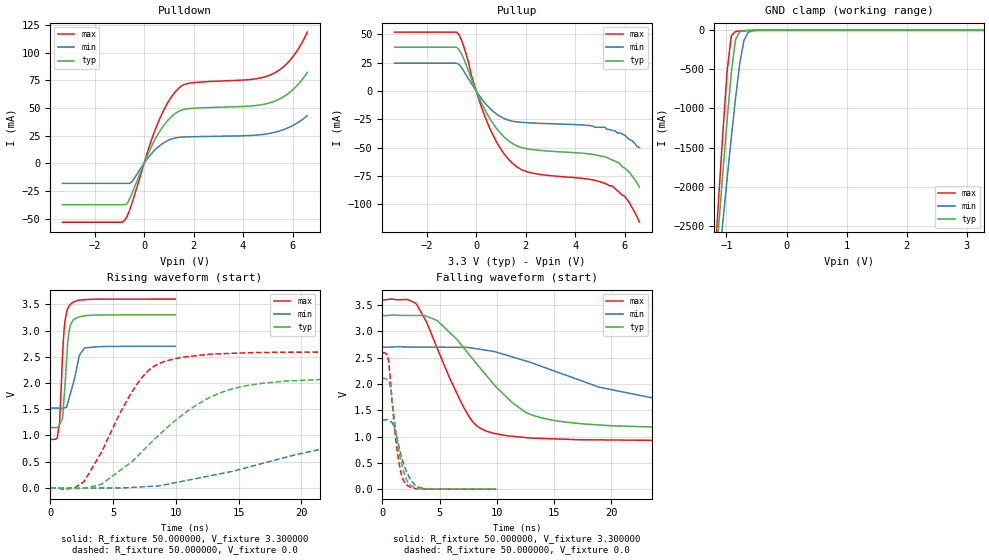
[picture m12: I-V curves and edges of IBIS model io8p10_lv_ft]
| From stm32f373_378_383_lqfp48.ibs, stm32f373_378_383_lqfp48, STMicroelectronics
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|   Model io8p10_lv_ft
[Model]  io8p10_lv_ft
Model_type I/O
Polarity   Non-Inverting
Enable   Active-Low
Vinl =   0.990000V
Vinh =   2.310000V
Vmeas =  1.650000V
Cref =   50.000000pF
Rref =   100.000000M
Vref =   0.0V
C_comp   5.028100pF   4.857200pF   5.254400pF
[Temperature Range]   25.000000   0.125000k   -40.000000
[Pullup Reference]   3.300000V   2.700000V   3.600000V
[Pulldown Reference]   0.0V   0.0V   0.0V
[POWER Clamp Reference]   3.300000V   2.700000V   3.600000V
[GND Clamp Reference]   0.0V   0.0V   0.0V
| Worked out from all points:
|   slope of the pulldown table from 0 to 0.495 V, typ, clamps not added: 20.9 ohm
|   slope of the pullup table from 0 to 0.495 V, typ, clamps not added: 22.2 ohm
|   GND clamp passes 1 mA (typ) near -0.59 V on its own axis
|   rising waveform, R_fixture 50.000000, V_fixture 3.300000: 20-80 % time 376ps typ, 706ps min, 340ps max; typ from 1.15 V to 3.3 V
|   rising waveform, R_fixture 50.000000, V_fixture 0.0: 20-80 % time 6.33ns typ, 15ns min, 3.53ns max; typ from 0 V to 2.1 V
|   falling waveform, R_fixture 50.000000, V_fixture 3.300000: 20-80 % time 5.37ns typ, 11ns min, 3.28ns max; typ from 3.3 V to 1.15 V
|   falling waveform, R_fixture 50.000000, V_fixture 0.0: 20-80 % time 885ps typ, 1.07ns min, 741ps max; typ from 2.1 V to 0 V
[Pulldown]
|Voltage   I(typ)   I(min)   I(max)
-3.3V     -37.45mA   -18.2mA    -53.24mA
-800mV    -37.45mA   -18.2mA    -51.9mA
-700mV    -36.7mA    -18.2mA    -48.48mA
-500mV    -27.71mA   -17.01mA   -36.66mA
200mV     10.57mA    6.084mA    14.57mA
500mV     23.91mA    13.38mA    33.24mA
900mV     37.17mA    19.87mA    52.48mA
1.3V      45.55mA    23.01mA    65.5mA
1.8V      49.29mA    23.83mA    72.18mA
5.1V      54.68mA    27.07mA    79.72mA
5.9V      64.2mA     32.82mA    93.01mA
6.6V      82.13mA    42.97mA    118.4mA
[Pullup]
|Voltage   I(typ)   I(min)   I(max)
-3.3V     38.73mA    24.6mA     52.09mA
-800mV    38.73mA    24.6mA     52.09mA
-500mV    28.38mA    17.49mA    39.19mA
0V        90fA       16pA       0A
500mV     -22.5mA    -14.16mA   -30.52mA
900mV     -35.28mA   -21.55mA   -48mA
1.4V      -45.54mA   -26.4mA    -62.53mA
2.2V      -51.57mA   -28.22mA   -72.25mA
4.7V      -56mA      -31mA      -78.6mA
5.5V      -61mA      -35mA      -84mA
6V        -68mA      -39mA      -93mA
6.6V      -85mA      -50mA      -116mA
[GND_clamp]
|Voltage   I(typ)   I(min)   I(max)
-3.3V     -9.706A    -9.438A    -9.292A
-1.2V     -3.211A    -3.571A    -3.02A
-1.13V    -2.511A    -3.008A    -2.153A
-1.06V    -1.824A    -2.453A    -1.311A
-990mV    -1.16A     -1.907A    -534mA
-920mV    -548mA     -1.377A    -70.08mA
-850mV    -120.4mA   -875.9mA   -15.9mA
-780mV    -17.66mA   -430.9mA   -9.191mA
-710mV    -5.44mA    -130.8mA   -5.02mA
-640mV    -2.077mA   -25.65mA   -2.003mA
-570mV    -540.4uA   -6.293mA   -433.9uA
3.28V     0A         0A         0A
[POWER_clamp]
|Voltage   I(typ)   I(min)   I(max)
-3.28V    0A         0A         0A
0V        0A         0A         0A
[Ramp]
| variable   typ   min   max
dV/dt_r  1.26234/6.32271n   0.77952/14.99025n   1.55460/3.52697n
dV/dt_f  1.28958/5.36294n   0.69804/10.97177n   1.60471/3.27728n
R_load = 50.000000
[Rising Waveform]
R_fixture= 50.000000
V_fixture= 3.300000
V_fixture_min= 2.700000
V_fixture_max= 3.600000
|time   V(typ)   V(min)   V(max)
0s        1.151V     1.522V     925.5mV
540.5ps   1.152V     1.522V     943.4mV
740.7ps   1.21V      1.521V     1.245V
981ps     1.324V     1.523V     2.536V
1.181ns   1.984V     1.53V      3.193V
1.401ns   2.808V     1.625V     3.426V
1.582ns   3.08V      1.78V      3.493V
2.322ns   3.26V      2.53V      3.578V
2.743ns   3.281V     2.668V     3.589V
9.97ns    3.3V       2.7V       3.6V
[Rising Waveform]
R_fixture= 50.000000
V_fixture= 0.0
V_fixture_min= 0.0
V_fixture_max= 0.0
|time   V(typ)   V(min)   V(max)
0s        -25.02uV   -17.47uV   -16.47uV
2.703ns   -1.021mV   -4.972mV   126.3mV
4.104ns   73.77mV    -631.6uV   691.1mV
7.307ns   691.9mV    21.61mV    2.105V
8.609ns   996.1mV    39.46mV    2.364V
10.41ns   1.37V      121.9mV    2.489V
13.61ns   1.82V      273.3mV    2.558V
18.82ns   2.037V     587.6mV    2.586V
30.13ns   2.101V     1.106V     2.591V
49.85ns   2.104V     1.316V     2.591V
[Falling Waveform]
R_fixture= 50.000000
V_fixture= 3.300000
V_fixture_min= 2.700000
V_fixture_max= 3.600000
|time   V(typ)   V(min)   V(max)
0s        3.3V       2.7V       3.6V
3.003ns   3.303V     2.701V     3.511V
4.805ns   3.203V     2.701V     2.673V
7.307ns   2.634V     2.697V     1.478V
8.308ns   2.367V     2.667V     1.195V
9.61ns    2.027V     2.623V     1.069V
12.61ns   1.449V     2.433V     979.4mV
17.32ns   1.245V     2.067V     939.9mV
24.02ns   1.18V      1.719V     928.2mV
49.85ns   1.151V     1.522V     925.5mV
[Falling Waveform]
R_fixture= 50.000000
V_fixture= 0.0
V_fixture_min= 0.0
V_fixture_max= 0.0
|time   V(typ)   V(min)   V(max)
0s        2.104V     1.316V     2.591V
500.5ps   2.07V      1.315V     2.49V
740.7ps   1.891V     1.283V     1.972V
1.001ns   1.436V     1.194V     1.301V
1.321ns   891.1mV    933.9mV    695.4mV
1.622ns   542mV      660.2mV    315.2mV
1.982ns   254.3mV    407.2mV    119.4mV
2.583ns   59.98mV    143.7mV    27.44mV
3.343ns   11.3mV     27.16mV    6.645mV
9.97ns    -25.02uV   -17.47uV   -16.47uV
